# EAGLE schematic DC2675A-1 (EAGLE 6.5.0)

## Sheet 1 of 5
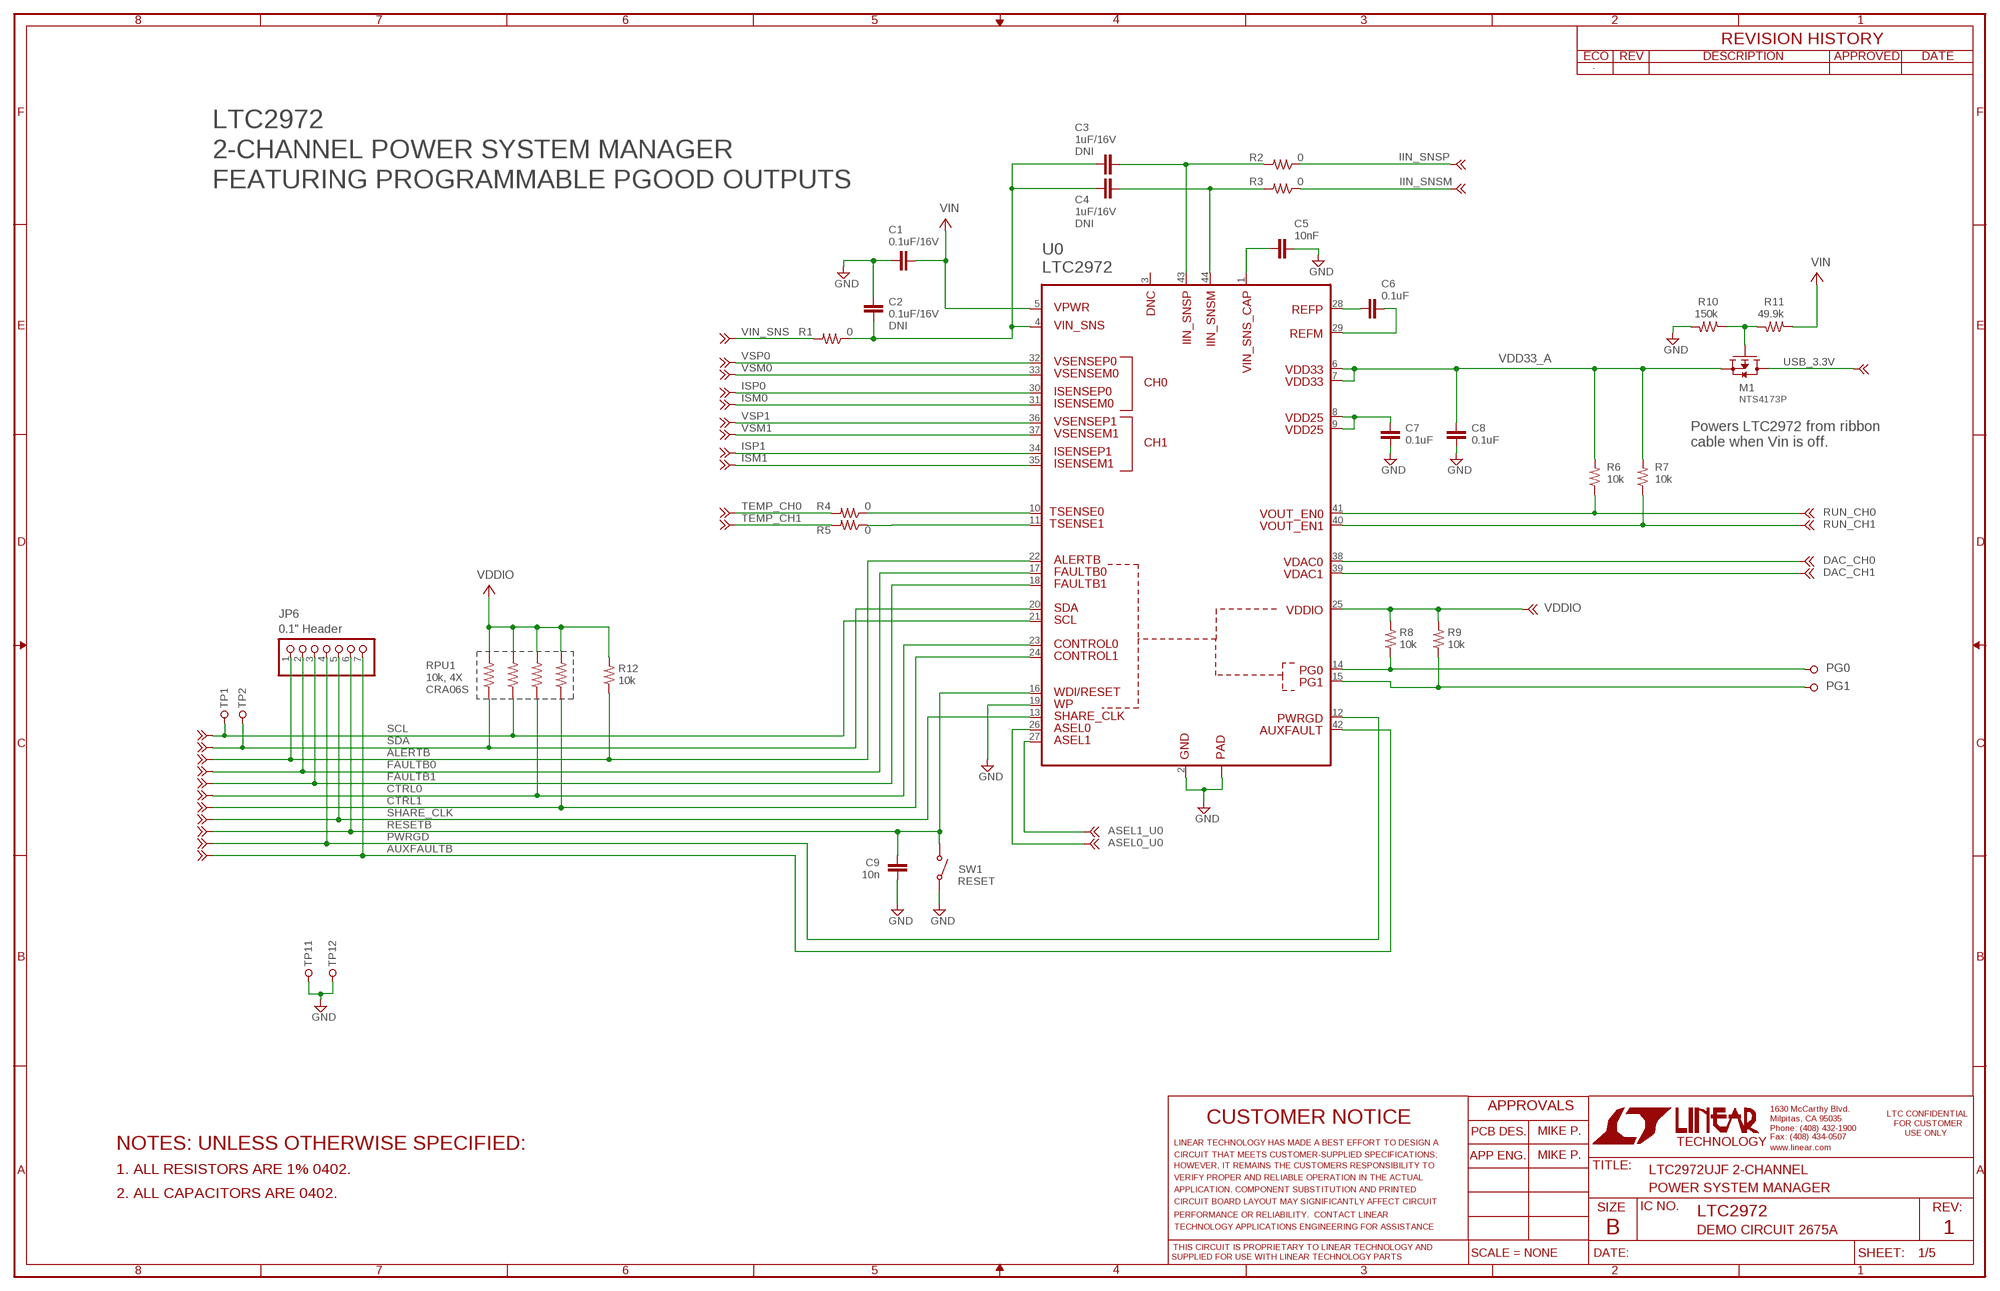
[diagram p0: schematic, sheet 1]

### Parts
C1  0.1uF/16V  CC0402  [C0402_BOX]
C2  0.1uF/16V  CC0402  [C0402_BOX]
C3  1uF/16V  CC0402  [C0402_BOX]
C4  1uF/16V  CC0402  [C0402_BOX]
C5  10nF  CC0402  [C0402_BOX]
C6  0.1uF  CC0402  [C0402_BOX]
C7  0.1uF  CC0402  [C0402_BOX]
C8  0.1uF  CC0402  [C0402_BOX]
C9  10n  CC0402  [C0402_BOX]
JP6  PINHD-1X7  [1X07]
M1  NTS4173P  PCH_SOT323  [SOT323]
R1  0  RR0402_BOX  [R0402_BOX]
R2  0  RR0402_BOX  [R0402_BOX]
R3  0  RR0402_BOX  [R0402_BOX]
R4  0  RR0402_BOX  [R0402_BOX]
R5  0  RR0402_BOX  [R0402_BOX]
R6  10k  RR0402_BOX  [R0402_BOX]
R7  10k  RR0402_BOX  [R0402_BOX]
R8  10k  RR0402_BOX  [R0402_BOX]
R9  10k  RR0402_BOX  [R0402_BOX]
R10  150k  RR0402_BOX  [R0402_BOX]
R11  49.9k  RR0402_BOX  [R0402_BOX]
R12  10k  RR0402_BOX  [R0402_BOX]
RPU1  10k, 4X  R_ARRAY_4X_CRA06S  [R_VISHAY_CRA06S]
SW1  PTS635SL25SMTR LFS  SWITCH_PTS635  [SWITCH_PTS635]
TP1  TURRET_SMALL_2308  [TURRET_SMALL_2308]
TP2  TURRET_SMALL_2308  [TURRET_SMALL_2308]
TP3  TURRET_SMALL_2308  [TURRET_SMALL_2308]
TP4  TURRET_SMALL_2308  [TURRET_SMALL_2308]
TP11  TURRET_SMALL_2308  [TURRET_SMALL_2308]
TP12  TURRET_SMALL_2308  [TURRET_SMALL_2308]
U0  LTC2972  [QFN44-6X7]

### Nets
ALERTB: JP6.1 R12.1 U0.22(ALERTB) ; also sheet 2,4,5
ASEL0_U0: U0.26(ASEL0) ; also sheet 3
ASEL1_U0: U0.27(ASEL1) ; also sheet 3
AUXFAULTB: JP6.7 U0.42(AUX_FAULT) ; also sheet 2,5
CTRL0: RPU1.R3_1 U0.23(CTRL0) ; also sheet 3,5
CTRL1: RPU1.R4_1 U0.24(CTRL1) ; also sheet 3,4,5
DAC_CH0: U0.38(VDAC0) ; also sheet 5
DAC_CH1: U0.39(VDAC1) ; also sheet 5
FAULTB0: JP6.2 U0.17(FAULTB0) ; also sheet 2,4,5
FAULTB1: JP6.3 U0.18(FAULTB1) ; also sheet 2,4,5
GND: C1.2 C2.1 C5.1 C7.2 C8.2 C9.1 R10.2 SW1.SW2 TP11.TP1 TP12.TP1 U0.2(GND) U0.19(WP) U0.45(PAD) ; also sheet 2,3,4,5
IIN_SNSM: R3.1 ; also sheet 5
IIN_SNSP: R2.1 ; also sheet 5
ISM0: U0.31(ISENSEM0) ; also sheet 3
ISM1: U0.35(ISENSEM1) ; also sheet 3
ISP0: U0.30(ISENSEP0) ; also sheet 3
ISP1: U0.34(ISENSEP1) ; also sheet 3
N$1: R4.1 U0.10(TSENSE0)
N$2: R5.1 U0.11(TSENSE1)
N$14: C2.2 C3.1 C4.1 R1.1 U0.4(VIN_SNS)
N$15: C3.2 R2.2 U0.43(IIN_SNSP)
N$16: C4.2 R3.2 U0.44(IIN_SNSM)
N$20: C5.2 U0.1(VIN_SNS_CAP)
N$48: C6.1 U0.28(REFP)
N$49: C6.2 U0.29(REFM)
N$52: C7.1 U0.8(VDD25) U0.9(VDD25)
PFET_GATE: M1.1(G) R10.1 R11.2 ; also sheet 2
PG0: R8.1 TP3.TP1 U0.14(PG0) ; also sheet 4
PG1: R9.1 TP4.TP1 U0.15(PG1) ; also sheet 4
PWRGD: JP6.4 U0.12(PWRGD) ; also sheet 2
RESETB: C9.2 JP6.6 SW1.SW1 U0.16(WDI-RESET) ; also sheet 2,5
RUN_CH0: R6.1 U0.41(VOUT_EN0) ; also sheet 5
RUN_CH1: R7.1 U0.40(VOUT_EN1) ; also sheet 5
SCL: RPU1.R2_1 TP1.TP1 U0.21(SCL) ; also sheet 2,5
SDA: RPU1.R1_1 TP2.TP1 U0.20(SDA) ; also sheet 2,5
SHARE_CLK: JP6.5 U0.13(SHARE_CLK) ; also sheet 2,5
TEMP_CH0: R4.2 ; also sheet 5
TEMP_CH1: R5.2 ; also sheet 5
USB_3.3V: M1.3(D) ; also sheet 2,5
VDD33_A: C8.1 M1.2(S) R6.2 R7.2 U0.6(VDD33) U0.7(VDD33) ; also sheet 3,4
VDDIO: R8.2 R9.2 R12.2 RPU1.R1_2 RPU1.R2_2 RPU1.R3_2 RPU1.R4_2 U0.25(VDDIO) ; also sheet 2,3,5
VIN: C1.1 R11.1 U0.5(VPWR) ; also sheet 2,5
VIN_SNS: R1.2 ; also sheet 2,5
VSM0: U0.33(VSENSEM0) ; also sheet 3
VSM1: U0.37(VSENSEM1) ; also sheet 3
VSP0: U0.32(VSENSEP0) ; also sheet 3
VSP1: U0.36(VSENSEP1) ; also sheet 3
Unconnected: U0.3(DNC)

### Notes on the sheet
- LTC2972
- 2-CHANNEL POWER SYSTEM MANAGER | DNI
- FEATURING PROGRAMMABLE PGOOD OUTPUTS
- DNI
- DNI
- Powers LTC2972 from ribbon
  cable when Vin is off.
- 0.1" Header
- CRA06S
- RESET
- MIKE P.
- NOTES: UNLESS OTHERWISE SPECIFIED:
- MIKE P.
- 1. ALL RESISTORS ARE 1% 0402. | LTC2972UJF 2-CHANNEL
- POWER SYSTEM MANAGER
- 2. ALL CAPACITORS ARE 0402.
- LTC2972
- DEMO CIRCUIT 2675A | 1

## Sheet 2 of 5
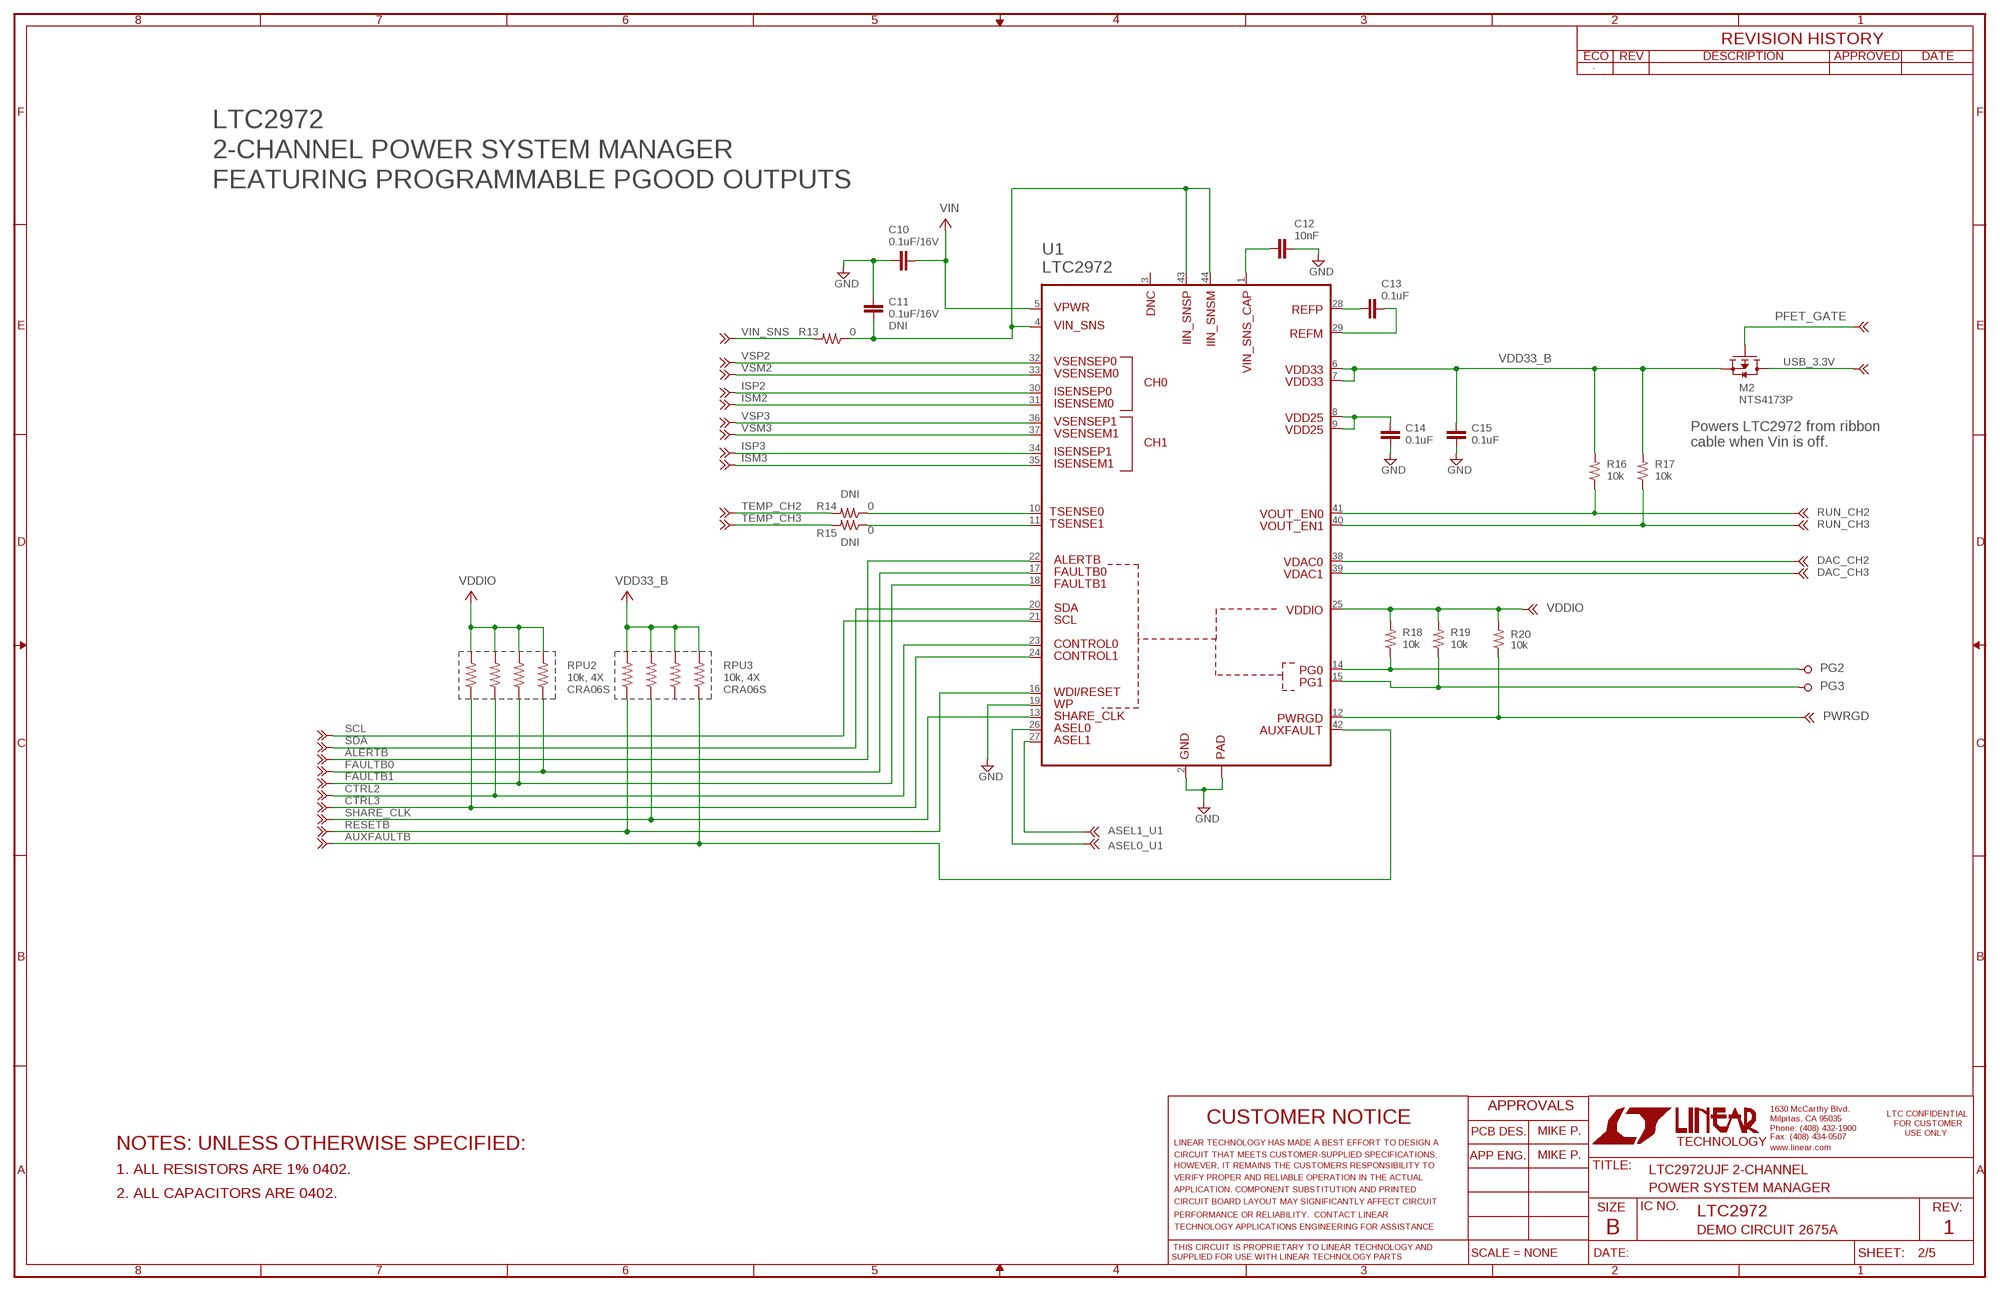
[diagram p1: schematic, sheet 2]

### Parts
C10  0.1uF/16V  CC0402  [C0402_BOX]
C11  0.1uF/16V  CC0402  [C0402_BOX]
C12  10nF  CC0402  [C0402_BOX]
C13  0.1uF  CC0402  [C0402_BOX]
C14  0.1uF  CC0402  [C0402_BOX]
C15  0.1uF  CC0402  [C0402_BOX]
M2  NTS4173P  PCH_SOT323  [SOT323]
R13  0  RR0402_BOX  [R0402_BOX]
R14  0  RR0402_BOX  [R0402_BOX]
R15  0  RR0402_BOX  [R0402_BOX]
R16  10k  RR0402_BOX  [R0402_BOX]
R17  10k  RR0402_BOX  [R0402_BOX]
R18  10k  RR0402_BOX  [R0402_BOX]
R19  10k  RR0402_BOX  [R0402_BOX]
R20  10k  RR0402_BOX  [R0402_BOX]
RPU2  10k, 4X  R_ARRAY_4X_CRA06S  [R_VISHAY_CRA06S]
RPU3  10k, 4X  R_ARRAY_4X_CRA06S  [R_VISHAY_CRA06S]
TP5  TURRET_SMALL_2308  [TURRET_SMALL_2308]
TP6  TURRET_SMALL_2308  [TURRET_SMALL_2308]
U1  LTC2972  [QFN44-6X7]

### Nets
ALERTB: U1.22(ALERTB) ; also sheet 1,4,5
ASEL0_U1: U1.26(ASEL0) ; also sheet 3
ASEL1_U1: U1.27(ASEL1) ; also sheet 3
AUXFAULTB: RPU3.R4_1 U1.42(AUX_FAULT) ; also sheet 1,5
CTRL2: RPU2.R2_1 U1.23(CTRL0) ; also sheet 3,4,5
CTRL3: RPU2.R1_1 U1.24(CTRL1) ; also sheet 3,4,5
DAC_CH2: U1.38(VDAC0) ; also sheet 5
DAC_CH3: U1.39(VDAC1) ; also sheet 5
FAULTB0: RPU2.R4_1 U1.17(FAULTB0) ; also sheet 1,4,5
FAULTB1: RPU2.R3_1 U1.18(FAULTB1) ; also sheet 1,4,5
GND: C10.2 C11.1 C12.1 C14.2 C15.2 U1.2(GND) U1.19(WP) U1.45(PAD) ; also sheet 1,3,4,5
ISM2: U1.31(ISENSEM0) ; also sheet 3
ISM3: U1.35(ISENSEM1) ; also sheet 3
ISP2: U1.30(ISENSEP0) ; also sheet 3
ISP3: U1.34(ISENSEP1) ; also sheet 3
N$4: R14.1 U1.10(TSENSE0)
N$5: R15.1 U1.11(TSENSE1)
N$17: C11.2 R13.1 U1.4(VIN_SNS) U1.43(IIN_SNSP) U1.44(IIN_SNSM)
N$24: C13.1 U1.28(REFP)
N$25: C13.2 U1.29(REFM)
N$26: C14.1 U1.8(VDD25) U1.9(VDD25)
N$27: C12.2 U1.1(VIN_SNS_CAP)
PFET_GATE: M2.1(G) ; also sheet 1
PG2: R18.1 TP5.TP1 U1.14(PG0) ; also sheet 4
PG3: R19.1 TP6.TP1 U1.15(PG1) ; also sheet 4
PWRGD: R20.1 U1.12(PWRGD) ; also sheet 1
RESETB: RPU3.R1_1 U1.16(WDI-RESET) ; also sheet 1,5
RUN_CH2: R16.1 U1.41(VOUT_EN0) ; also sheet 5
RUN_CH3: R17.1 U1.40(VOUT_EN1) ; also sheet 5
SCL: U1.21(SCL) ; also sheet 1,5
SDA: U1.20(SDA) ; also sheet 1,5
SHARE_CLK: RPU3.R2_1 U1.13(SHARE_CLK) ; also sheet 1,5
TEMP_CH2: R14.2 ; also sheet 5
TEMP_CH3: R15.2 ; also sheet 5
USB_3.3V: M2.3(D) ; also sheet 1,5
VDD33_B: C15.1 M2.2(S) R16.2 R17.2 RPU3.R1_2 RPU3.R2_2 RPU3.R3_2 RPU3.R4_2 U1.6(VDD33) U1.7(VDD33) ; also sheet 3,4,5
VDDIO: R18.2 R19.2 R20.2 RPU2.R1_2 RPU2.R2_2 RPU2.R3_2 RPU2.R4_2 U1.25(VDDIO) ; also sheet 1,3,5
VIN: C10.1 U1.5(VPWR) ; also sheet 1,5
VIN_SNS: R13.2 ; also sheet 1,5
VSM2: U1.33(VSENSEM0) ; also sheet 3
VSM3: U1.37(VSENSEM1) ; also sheet 3
VSP2: U1.32(VSENSEP0) ; also sheet 3
VSP3: U1.36(VSENSEP1) ; also sheet 3
Unconnected: RPU3.R3_1 U1.3(DNC)

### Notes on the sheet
- LTC2972
- 2-CHANNEL POWER SYSTEM MANAGER
- FEATURING PROGRAMMABLE PGOOD OUTPUTS
- DNI
- Powers LTC2972 from ribbon
  cable when Vin is off.
- DNI
- DNI
- CRA06S | CRA06S
- MIKE P.
- NOTES: UNLESS OTHERWISE SPECIFIED:
- MIKE P.
- 1. ALL RESISTORS ARE 1% 0402. | LTC2972UJF 2-CHANNEL
- POWER SYSTEM MANAGER
- 2. ALL CAPACITORS ARE 0402.
- LTC2972
- DEMO CIRCUIT 2675A | 1

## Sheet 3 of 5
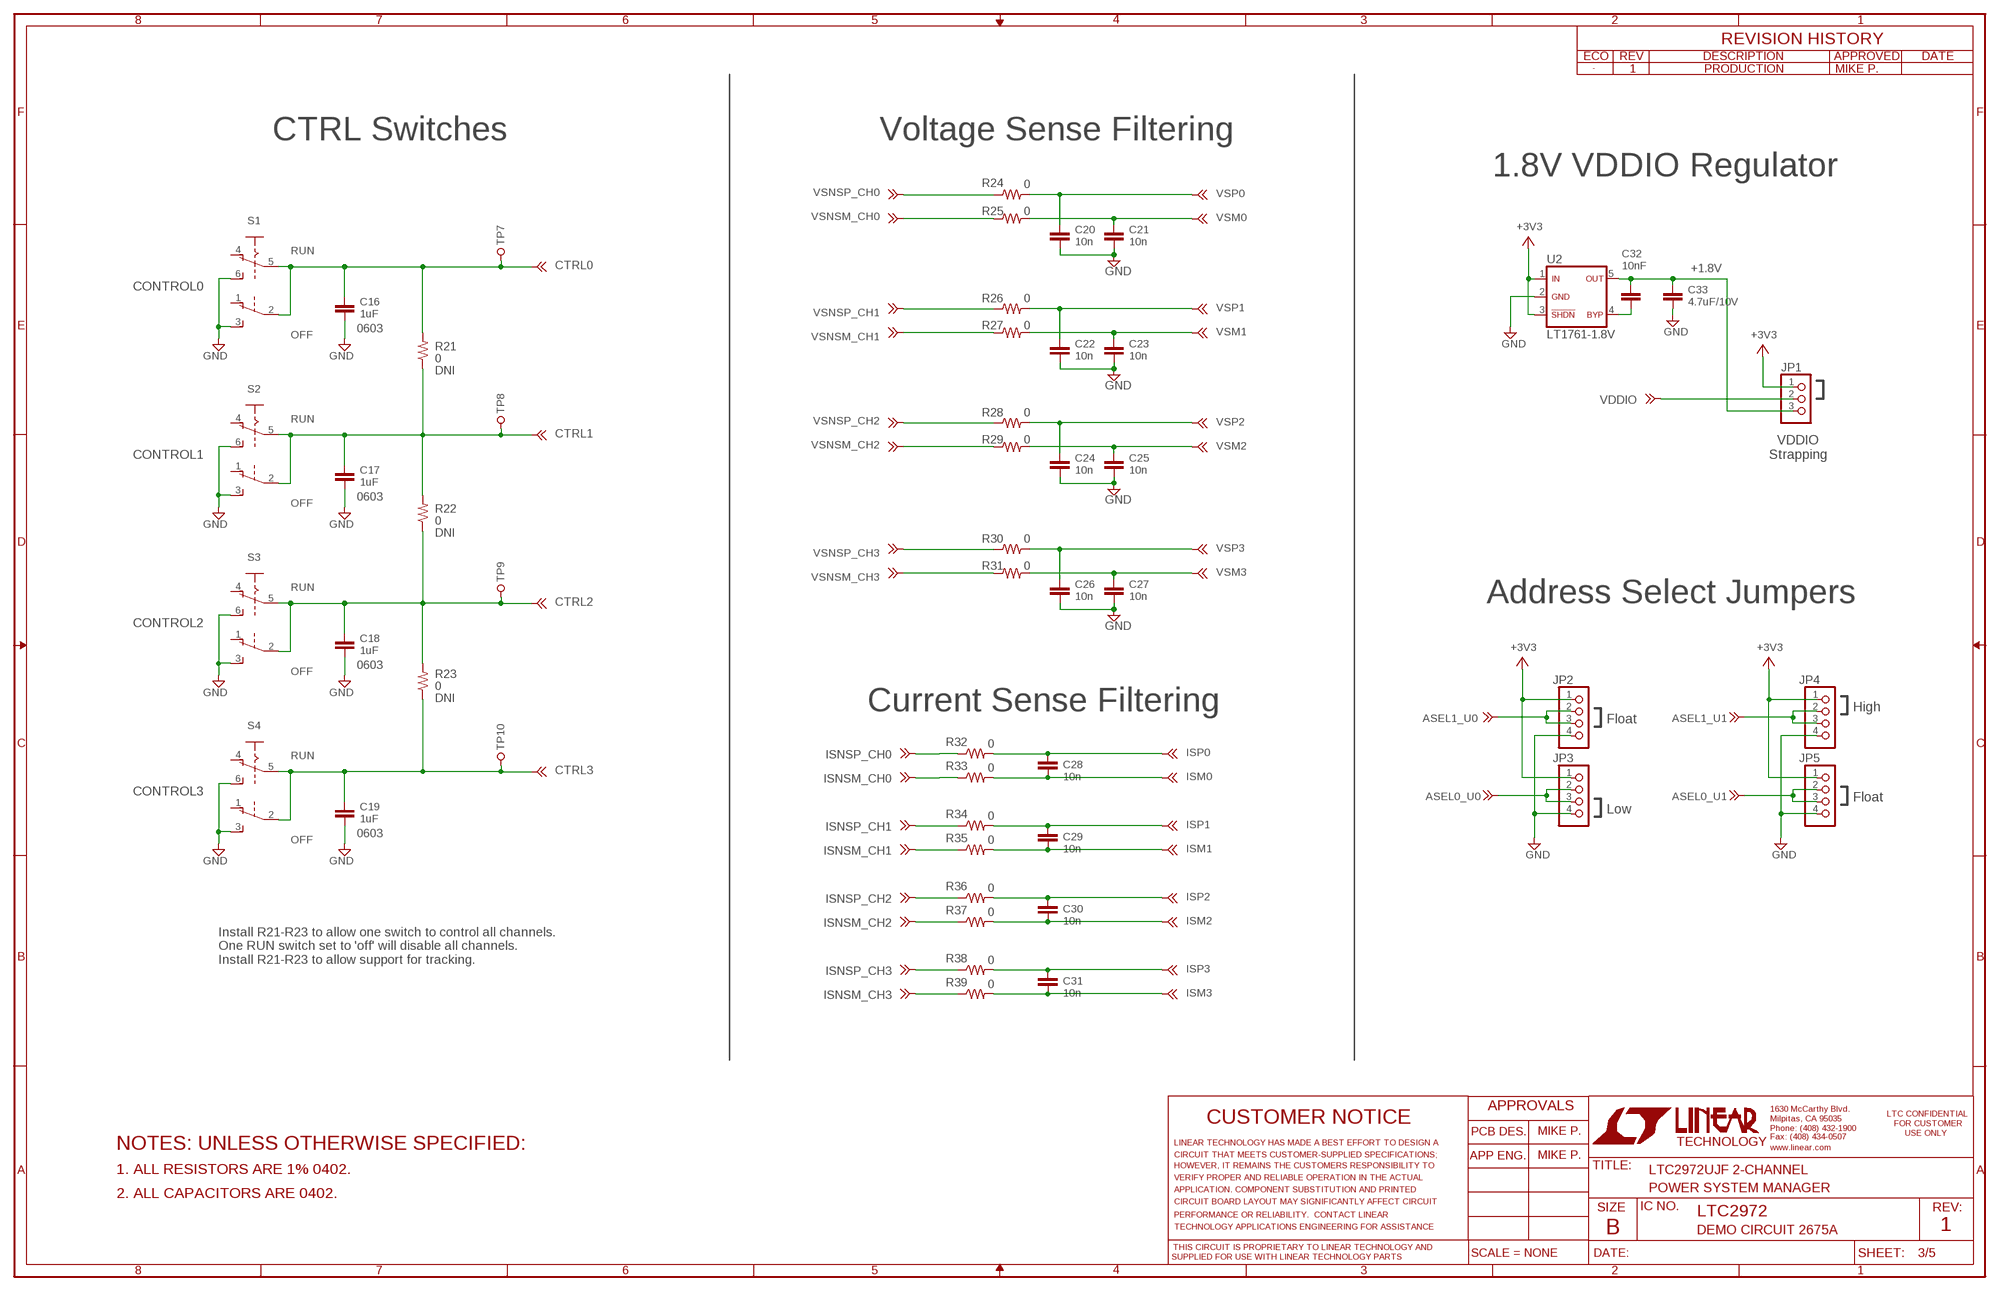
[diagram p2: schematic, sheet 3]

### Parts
C16  1uF  CC0603_BOX  [C0603_BOX]
C17  1uF  CC0603_BOX  [C0603_BOX]
C18  1uF  CC0603_BOX  [C0603_BOX]
C19  1uF  CC0603_BOX  [C0603_BOX]
C20  10n  CC0402  [C0402_BOX]
C21  10n  CC0402  [C0402_BOX]
C22  10n  CC0402  [C0402_BOX]
C23  10n  CC0402  [C0402_BOX]
C24  10n  CC0402  [C0402_BOX]
C25  10n  CC0402  [C0402_BOX]
C26  10n  CC0402  [C0402_BOX]
C27  10n  CC0402  [C0402_BOX]
C28  10n  CC0402  [C0402_BOX]
C29  10n  CC0402  [C0402_BOX]
C30  10n  CC0402  [C0402_BOX]
C31  10n  CC0402  [C0402_BOX]
C32  10nF  CC0402  [C0402_BOX]
C33  4.7uF/10V  CC0402  [C0402_BOX]
JP1  PINHD-1X3-2MM  [1X03-2MM]
JP2  PINHD-1X4-2MM  [1X04-2MM]
JP3  PINHD-1X4-2MM  [1X04-2MM]
JP4  PINHD-1X4-2MM  [1X04-2MM]
JP5  PINHD-1X4-2MM  [1X04-2MM]
R21  0  RR0402_BOX  [R0402_BOX]
R22  0  RR0402_BOX  [R0402_BOX]
R23  0  RR0402_BOX  [R0402_BOX]
R24  0  RR0402_BOX  [R0402_BOX]
R25  0  RR0402_BOX  [R0402_BOX]
R26  0  RR0402_BOX  [R0402_BOX]
R27  0  RR0402_BOX  [R0402_BOX]
R28  0  RR0402_BOX  [R0402_BOX]
R29  0  RR0402_BOX  [R0402_BOX]
R30  0  RR0402_BOX  [R0402_BOX]
R31  0  RR0402_BOX  [R0402_BOX]
R32  0  RR0402_BOX  [R0402_BOX]
R33  0  RR0402_BOX  [R0402_BOX]
R34  0  RR0402_BOX  [R0402_BOX]
R35  0  RR0402_BOX  [R0402_BOX]
R36  0  RR0402_BOX  [R0402_BOX]
R37  0  RR0402_BOX  [R0402_BOX]
R38  0  RR0402_BOX  [R0402_BOX]
R39  0  RR0402_BOX  [R0402_BOX]
S1  CONTROL0  JS202011CQN  [JS202011CQN]
S2  CONTROL1  JS202011CQN  [JS202011CQN]
S3  CONTROL2  JS202011CQN  [JS202011CQN]
S4  CONTROL3  JS202011CQN  [JS202011CQN]
TP7  TURRET_SMALL_2308  [TURRET_SMALL_2308]
TP8  TURRET_SMALL_2308  [TURRET_SMALL_2308]
TP9  TURRET_SMALL_2308  [TURRET_SMALL_2308]
TP10  TURRET_SMALL_2308  [TURRET_SMALL_2308]
U2  LT1761-1.8V  LT1761-X  [SOT-23-5]

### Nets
1V8: C32.1 C33.1 JP1.3 U2.5(OUT)
ASEL0_U0: JP3.2 JP3.3 ; also sheet 1
ASEL0_U1: JP5.2 JP5.3 ; also sheet 2
ASEL1_U0: JP2.2 JP2.3 ; also sheet 1
ASEL1_U1: JP4.2 JP4.3 ; also sheet 2
CTRL0: C16.1 R21.2 S1.2(B:P) S1.5(A:P) TP7.TP1 ; also sheet 1,5
CTRL1: C17.1 R21.1 R22.2 S2.2(B:P) S2.5(A:P) TP8.TP1 ; also sheet 1,4,5
CTRL2: C18.1 R22.1 R23.2 S3.2(B:P) S3.5(A:P) TP9.TP1 ; also sheet 2,4,5
CTRL3: C19.1 R23.1 S4.2(B:P) S4.5(A:P) TP10.TP1 ; also sheet 2,4,5
GND: C16.2 C17.2 C18.2 C19.2 C20.2 C21.2 C22.2 C23.2 C24.2 C25.2 C26.2 C27.2 C33.2 JP2.4 JP3.4 JP4.4 JP5.4 S1.3(B:S) S1.6(A:S) S2.3(B:S) S2.6(A:S) S3.3(B:S) S3.6(A:S) S4.3(B:S) S4.6(A:S) U2.2(GND) ; also sheet 1,2,4,5
ISM0: C28.2 R33.2 ; also sheet 1
ISM1: C29.2 R35.2 ; also sheet 1
ISM2: C30.2 R37.2 ; also sheet 2
ISM3: C31.2 R39.2 ; also sheet 2
ISNSM_CH0: R33.1 ; also sheet 5
ISNSM_CH1: R35.1 ; also sheet 5
ISNSM_CH2: R37.1 ; also sheet 5
ISNSM_CH3: R39.1 ; also sheet 5
ISNSP_CH0: R32.1 ; also sheet 5
ISNSP_CH1: R34.1 ; also sheet 5
ISNSP_CH2: R36.1 ; also sheet 5
ISNSP_CH3: R38.1 ; also sheet 5
ISP0: C28.1 R32.2 ; also sheet 1
ISP1: C29.1 R34.2 ; also sheet 1
ISP2: C30.1 R36.2 ; also sheet 2
ISP3: C31.1 R38.2 ; also sheet 2
N$34: C32.2 U2.4(BYP)
VDD33_A: JP1.1 JP2.1 JP3.1 U2.1(IN) U2.3(SHDN) ; supply symbol labelled +3V3 ; also sheet 1,4
VDD33_B: JP4.1 JP5.1 ; supply symbol labelled +3V3 ; also sheet 2,4,5
VDDIO: JP1.2 ; also sheet 1,2,5
VSM0: C21.1 R25.2 ; also sheet 1
VSM1: C23.1 R27.2 ; also sheet 1
VSM2: C25.1 R29.2 ; also sheet 2
VSM3: C27.1 R31.2 ; also sheet 2
VSNSM_CH0: R25.1 ; also sheet 5
VSNSM_CH1: R27.1 ; also sheet 5
VSNSM_CH2: R29.1 ; also sheet 5
VSNSM_CH3: R31.1 ; also sheet 5
VSNSP_CH0: R24.1 ; also sheet 5
VSNSP_CH1: R26.1 ; also sheet 5
VSNSP_CH2: R28.1 ; also sheet 5
VSNSP_CH3: R30.1 ; also sheet 5
VSP0: C20.1 R24.2 ; also sheet 1
VSP1: C22.1 R26.2 ; also sheet 1
VSP2: C24.1 R28.2 ; also sheet 2
VSP3: C26.1 R30.2 ; also sheet 2
Unconnected: S1.1(B:O) S1.4(A:O) S2.1(B:O) S2.4(A:O) S3.1(B:O) S3.4(A:O) S4.1(B:O) S4.4(A:O)

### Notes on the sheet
- 1 | PRODUCTION | MIKE P.
- CTRL Switches | Voltage Sense Filtering
- 1.8V VDDIO Regulator
- RUN
- +1.8V
- 0603
- OFF
- DNI
- RUN
- VDDIO
  Strapping
- 0603
- OFF
- DNI
- RUN
- Address Select Jumpers
- 0603
- OFF
- DNI
- Current Sense Filtering | High
- Float
- RUN
- Float
- Low
- 0603
- OFF
- Install R21-R23 to allow one switch to control all channels.
  One RUN switch set to 'off' will disable all channels.
  Install R21-R23 to allow support for tracking.
- MIKE P.
- NOTES: UNLESS OTHERWISE SPECIFIED:
- MIKE P.
- 1. ALL RESISTORS ARE 1% 0402. | LTC2972UJF 2-CHANNEL
- POWER SYSTEM MANAGER
- 2. ALL CAPACITORS ARE 0402.
- LTC2972
- DEMO CIRCUIT 2675A | 1

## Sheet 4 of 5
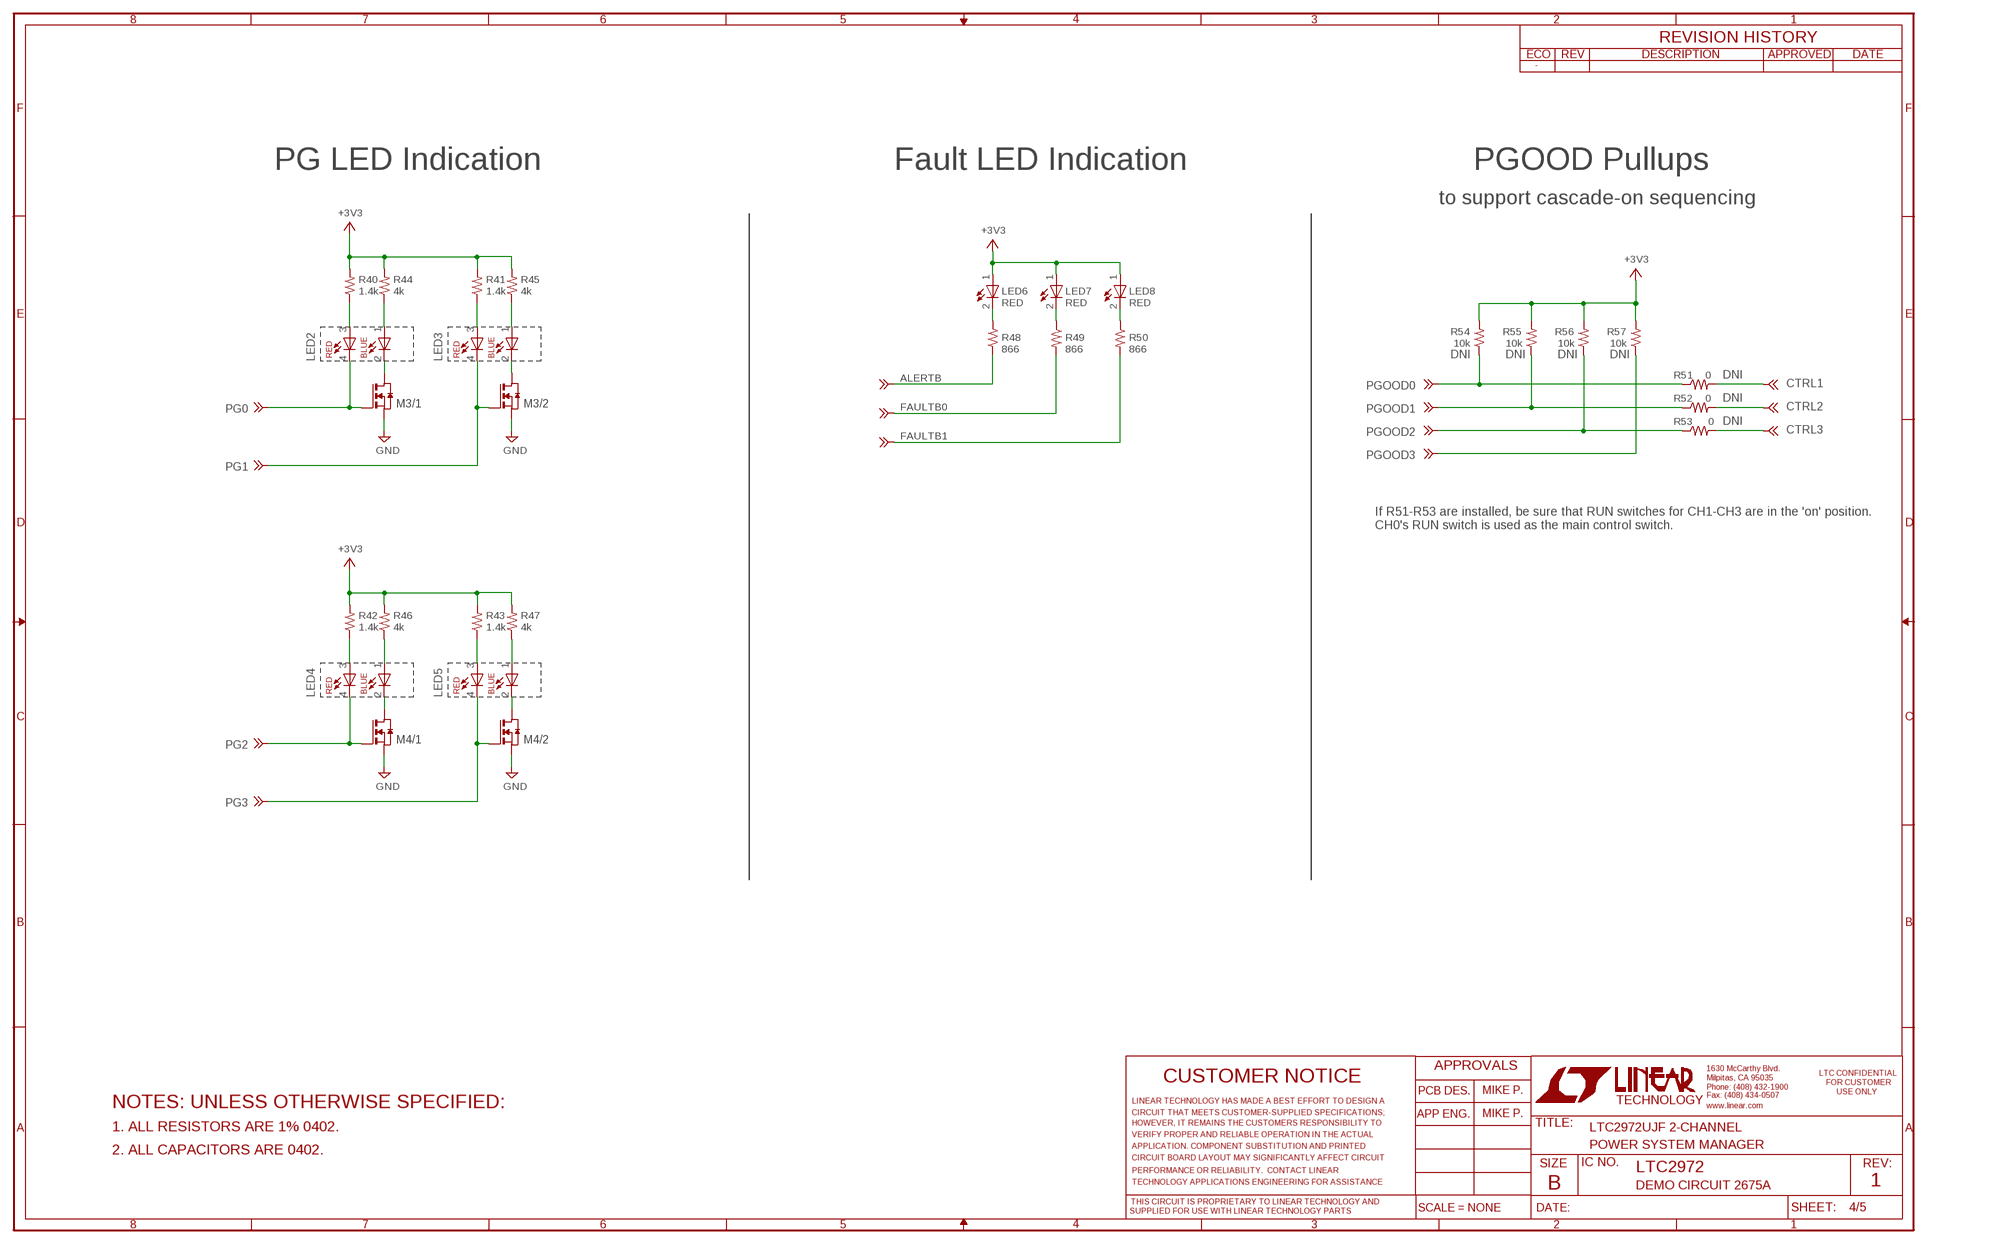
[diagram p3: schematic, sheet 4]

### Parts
LED2  Kingbright  LED-DUAL-COLOR_1.6X0.8MM  [LED-DUAL_1.6X0.8MM]
LED3  Kingbright  LED-DUAL-COLOR_1.6X0.8MM  [LED-DUAL_1.6X0.8MM]
LED4  Kingbright  LED-DUAL-COLOR_1.6X0.8MM  [LED-DUAL_1.6X0.8MM]
LED5  Kingbright  LED-DUAL-COLOR_1.6X0.8MM  [LED-DUAL_1.6X0.8MM]
LED6  RED  LED-0603  [CHIPLED_0603]
LED7  RED  LED-0603  [CHIPLED_0603]
LED8  RED  LED-0603  [CHIPLED_0603]
M3  NCH_DUAL_REVERSE  [SOT-363]
M4  NCH_DUAL_REVERSE  [SOT-363]
R40  1.4k  RR0402_BOX  [R0402_BOX]
R41  1.4k  RR0402_BOX  [R0402_BOX]
R42  1.4k  RR0402_BOX  [R0402_BOX]
R43  1.4k  RR0402_BOX  [R0402_BOX]
R44  4k  RR0402_BOX  [R0402_BOX]
R45  4k  RR0402_BOX  [R0402_BOX]
R46  4k  RR0402_BOX  [R0402_BOX]
R47  4k  RR0402_BOX  [R0402_BOX]
R48  866  RR0402_BOX  [R0402_BOX]
R49  866  RR0402_BOX  [R0402_BOX]
R50  866  RR0402_BOX  [R0402_BOX]
R51  0  RR0402_BOX  [R0402_BOX]
R52  0  RR0402_BOX  [R0402_BOX]
R53  0  RR0402_BOX  [R0402_BOX]
R54  10k  RR0402_BOX  [R0402_BOX]
R55  10k  RR0402_BOX  [R0402_BOX]
R56  10k  RR0402_BOX  [R0402_BOX]
R57  10k  RR0402_BOX  [R0402_BOX]

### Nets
ALERTB: R48.1 ; also sheet 1,2,5
CTRL1: R51.2 ; also sheet 1,3,5
CTRL2: R52.2 ; also sheet 2,3,5
CTRL3: R53.2 ; also sheet 2,3,5
FAULTB0: R49.2 ; also sheet 1,2,5
FAULTB1: R50.2 ; also sheet 1,2,5
GND: M3.1(/1:S) M3.4(/2:S) M4.1(/1:S) M4.4(/2:S) ; also sheet 1,2,3,5
N$8: LED5.2(C2) M4.3(/2:D)
N$9: LED4.2(C2) M4.6(/1:D)
N$10: LED2.2(C2) M3.6(/1:D)
N$11: LED3.2(C2) M3.3(/2:D)
N$12: LED2.1(A1) R44.1
N$13: LED3.1(A1) R45.1
N$18: LED4.1(A1) R46.1
N$19: LED5.1(A1) R47.1
N$28: LED8.N(C) R50.1
N$29: LED7.N(C) R49.1
N$30: LED6.N(C) R48.2
N$36: LED2.3(A3) R40.1
N$42: LED3.3(A3) R41.1
N$56: LED4.3(A3) R42.1
N$83: LED5.3(A3) R43.1
PG0: LED2.4(C4) M3.2(/1:G) ; also sheet 1
PG1: LED3.4(C4) M3.5(/2:G) ; also sheet 1
PG2: LED4.4(C4) M4.2(/1:G) ; also sheet 2
PG3: LED5.4(C4) M4.5(/2:G) ; also sheet 2
PGOOD0: R51.1 R54.1 ; also sheet 5
PGOOD1: R52.1 R55.1 ; also sheet 5
PGOOD2: R53.1 R56.1 ; also sheet 5
PGOOD3: R57.1 ; also sheet 5
VDD33_A: R40.2 R41.2 R44.2 R45.2 ; supply symbol labelled +3V3 ; also sheet 1,3
VDD33_B: LED6.P(A) LED7.P(A) LED8.P(A) R42.2 R43.2 R46.2 R47.2 R54.2 R55.2 R56.2 R57.2 ; supply symbol labelled +3V3 ; also sheet 2,3,5

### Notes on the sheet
- PG LED Indication | Fault LED Indication | PGOOD Pullups
- to support cascade-on sequencing
- DNI | DNI | DNI | DNI
- DNI
- DNI
- DNI
- If R51-R53 are installed, be sure that RUN switches for CH1-CH3 are in the 'on' position.
  CH0's RUN switch is used as the main control switch.
- MIKE P.
- NOTES: UNLESS OTHERWISE SPECIFIED:
- MIKE P.
- 1. ALL RESISTORS ARE 1% 0402. | LTC2972UJF 2-CHANNEL
- POWER SYSTEM MANAGER
- 2. ALL CAPACITORS ARE 0402.
- LTC2972
- DEMO CIRCUIT 2675A | 1

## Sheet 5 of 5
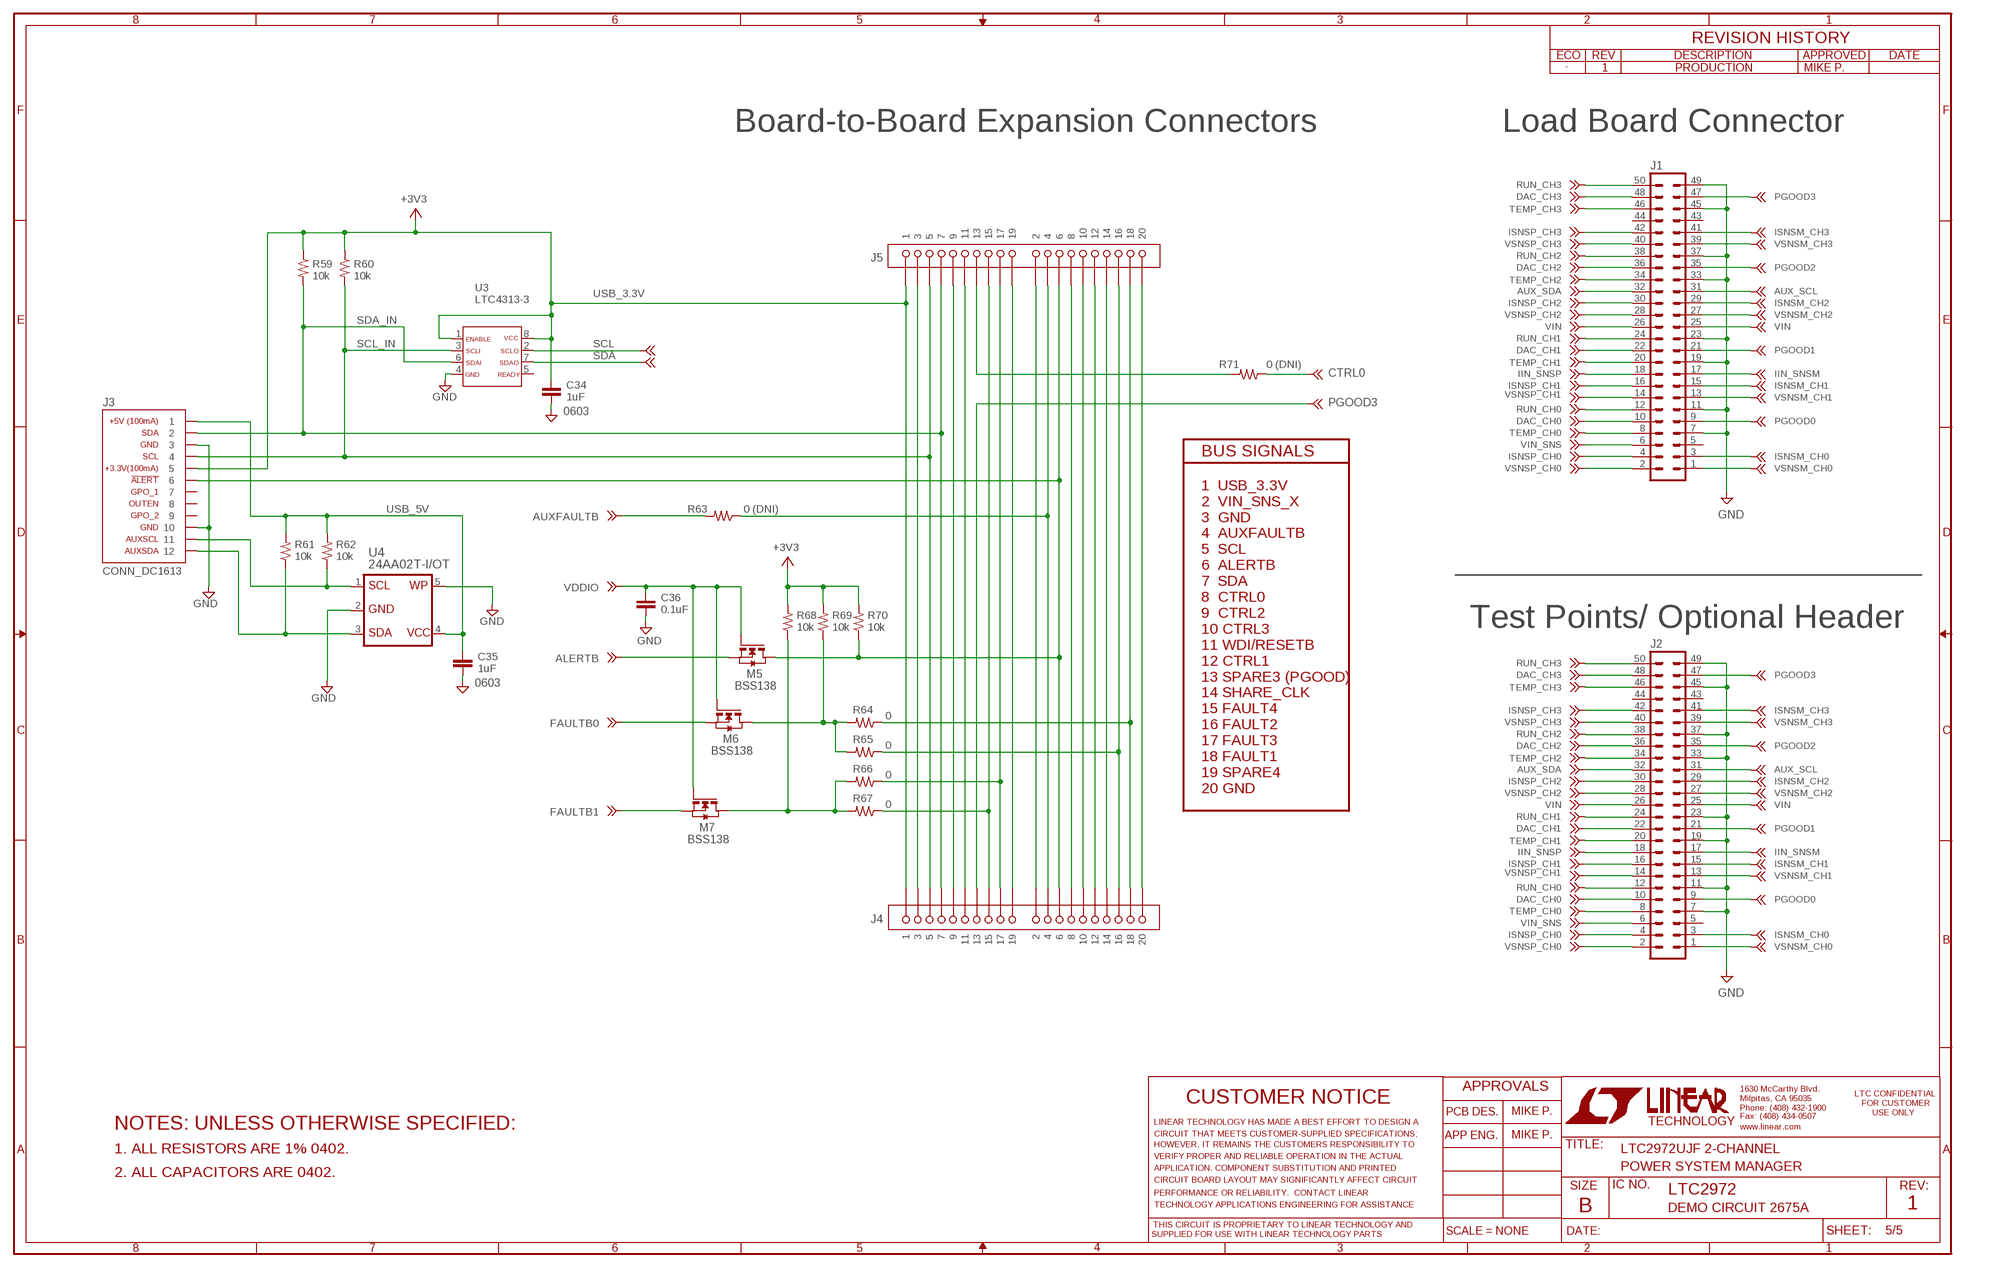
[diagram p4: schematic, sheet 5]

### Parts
C34  1uF  CC0603_BOX  [C0603_BOX]
C35  1uF  CC0603_BOX  [C0603_BOX]
C36  0.1uF  CC0402  [C0402_BOX]
J1  CONN_2X25_RECEPT  [PINHEAD_2X25_RECEPT]
J2  CONN_2X25_RECEPT_NO_SILK  [PINHEAD_2X25_RECEPT_NO_SILK]
J3  CONN_DC1613  [CONN_DC1613]
J4  HEADER_CONN_2X10_0.1INCH  [HEADER_2X10_0.1INCH]
J5  RECEPT_CONN_2X10_0.1INCH  [RECEPT_2X10_0.1INCH]
M5  BSS138  NCH_SOT23  [SOT23]
M6  BSS138  NCH_SOT23  [SOT23]
M7  BSS138  NCH_SOT23  [SOT23]
R59  10k  RR0402_BOX  [R0402_BOX]
R60  10k  RR0402_BOX  [R0402_BOX]
R61  10k  RR0402_BOX  [R0402_BOX]
R62  10k  RR0402_BOX  [R0402_BOX]
R63  0 (DNI)  RR0402_BOX  [R0402_BOX]
R64  0  RR0402_BOX  [R0402_BOX]
R65  0  RR0402_BOX  [R0402_BOX]
R66  0  RR0402_BOX  [R0402_BOX]
R67  0  RR0402_BOX  [R0402_BOX]
R68  10k  RR0402_BOX  [R0402_BOX]
R69  10k  RR0402_BOX  [R0402_BOX]
R70  10k  RR0402_BOX  [R0402_BOX]
R71  0 (DNI)  RR0402_BOX  [R0402_BOX]
U3  LTC4313-3  LTC4313_MS8  [MSOP-8]
U4  24AA02T-I/OT  24AA64  [SOT-23-5]

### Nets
ALERTB: M5.2(S) ; also sheet 1,2,4
ALERTB_3V3: J3.6 J4.P$6 J5.P$6 M5.3(D) R70.1
AUX_SCL: J1.31 J2.31 J3.11 R62.1 U4.1
AUX_SDA: J1.32 J2.32 J3.12 R61.1 U4.3
AUXFAULTB: R63.2 ; also sheet 1,2
AUXFAULTB_3V3: J4.P$4 J5.P$4 R63.1
CTRL0: J4.P$8 J5.P$8 R71.1 ; also sheet 1,3
CTRL1: J4.P$12 J5.P$12 ; also sheet 1,3,4
CTRL2: J4.P$9 J5.P$9 ; also sheet 2,3,4
CTRL3: J4.P$10 J5.P$10 ; also sheet 2,3,4
DAC_CH0: J1.10 J2.10 ; also sheet 1
DAC_CH1: J1.22 J2.22 ; also sheet 1
DAC_CH2: J1.36 J2.36 ; also sheet 2
DAC_CH3: J1.48 J2.48 ; also sheet 2
FAULT1: J4.P$18 J5.P$18 R64.1
FAULT2: J4.P$16 J5.P$16 R65.1
FAULT3: J4.P$17 J5.P$17 R66.1
FAULT4: J4.P$15 J5.P$15 R67.1
FAULTB0: M6.2(S) ; also sheet 1,2,4
FAULTB1: M7.2(S) ; also sheet 1,2,4
GND: C34.2 C35.2 C36.2 J1.7 J1.11 J1.19 J1.23 J1.33 J1.37 J1.45 J1.49 J2.7 J2.11 J2.19 J2.23 J2.33 J2.37 J2.45 J2.49 J3.3 J3.10 J4.P$3 J4.P$20 J5.P$3 J5.P$20 U3.4(GND) U4.2 U4.5 ; also sheet 1,2,3,4
IIN_SNSM: J1.17 J2.17 ; also sheet 1
IIN_SNSP: J1.18 J2.18 ; also sheet 1
ISNSM_CH0: J1.3 J2.3 ; also sheet 3
ISNSM_CH1: J1.15 J2.15 ; also sheet 3
ISNSM_CH2: J1.29 J2.29 ; also sheet 3
ISNSM_CH3: J1.41 J2.41 ; also sheet 3
ISNSP_CH0: J1.4 J2.4 ; also sheet 3
ISNSP_CH1: J1.16 J2.16 ; also sheet 3
ISNSP_CH2: J1.30 J2.30 ; also sheet 3
ISNSP_CH3: J1.42 J2.42 ; also sheet 3
N$6: J5.P$13 R71.2
N$21: M7.3(D) R66.2 R67.2 R68.1
N$23: M6.3(D) R64.2 R65.2 R69.1
PGOOD0: J1.9 J2.9 ; also sheet 4
PGOOD1: J1.21 J2.21 ; also sheet 4
PGOOD2: J1.35 J2.35 ; also sheet 4
PGOOD3: J1.47 J2.47 J4.P$13 ; also sheet 4
RESETB: J4.P$11 J5.P$11 ; also sheet 1,2
RUN_CH0: J1.12 J2.12 ; also sheet 1
RUN_CH1: J1.24 J2.24 ; also sheet 1
RUN_CH2: J1.38 J2.38 ; also sheet 2
RUN_CH3: J1.50 J2.50 ; also sheet 2
SCL: U3.2(SCLO) ; also sheet 1,2
SCL_IN: J3.4 J4.P$5 J5.P$5 R60.2 U3.3(SCLI)
SDA: U3.7(SDAO) ; also sheet 1,2
SDA_IN: J3.2 J4.P$7 J5.P$7 R59.2 U3.6(SDAI)
SHARE_CLK: J4.P$14 J5.P$14 ; also sheet 1,2
SPARE4: J4.P$19 J5.P$19
TEMP_CH0: J1.8 J2.8 ; also sheet 1
TEMP_CH1: J1.20 J2.20 ; also sheet 1
TEMP_CH2: J1.34 J2.34 ; also sheet 2
TEMP_CH3: J1.46 J2.46 ; also sheet 2
USB_3.3V: C34.1 J3.5 J4.P$1 J5.P$1 R59.1 R60.1 U3.1(EN) U3.8(VCC) ; supply symbol labelled +3V3 ; also sheet 1,2
USB_5V: C35.1 J3.1 R61.2 R62.2 U4.4
VDD33_B: R68.2 R69.2 R70.2 ; supply symbol labelled +3V3 ; also sheet 2,3,4
VDDIO: C36.1 M5.1(G) M6.1(G) M7.1(G) ; also sheet 1,2,3
VIN: J1.25 J1.26 J2.25 J2.26 ; also sheet 1,2
VIN_SNS: J1.6 J2.6 ; also sheet 1,2
VIN_SNS_X: J4.P$2 J5.P$2
VSNSM_CH0: J1.1 J2.1 ; also sheet 3
VSNSM_CH1: J1.13 J2.13 ; also sheet 3
VSNSM_CH2: J1.27 J2.27 ; also sheet 3
VSNSM_CH3: J1.39 J2.39 ; also sheet 3
VSNSP_CH0: J1.2 J2.2 ; also sheet 3
VSNSP_CH1: J1.14 J2.14 ; also sheet 3
VSNSP_CH2: J1.28 J2.28 ; also sheet 3
VSNSP_CH3: J1.40 J2.40 ; also sheet 3
Unconnected: J1.5 J1.43 J1.44 J2.5 J2.43 J2.44 J3.7 J3.8 J3.9 U3.5(RDY)

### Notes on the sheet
- 1 | PRODUCTION | MIKE P.
- Board-to-Board Expansion Connectors | Load Board Connector
- 0603
- VIN_SNS
- BUS SIGNALS
- Test Points/ Optional Header
- 0603
- 1  USB_3.3V
  2  VIN_SNS_X
  3  GND
  4  AUXFAULTB
  5  SCL
  6  ALERTB
  7  SDA
  8  CTRL0
  9  CTRL2
  10 CTRL3
  11 WDI/RESETB
  12 CTRL1
  13 SPARE3 (PGOOD)
  14 SHARE_CLK
  15 FAULT4
  16 FAULT2
  17 FAULT3
  18 FAULT1
  19 SPARE4
  20 GND
- VIN_SNS
- MIKE P.
- NOTES: UNLESS OTHERWISE SPECIFIED:
- MIKE P.
- 1. ALL RESISTORS ARE 1% 0402. | LTC2972UJF 2-CHANNEL
- POWER SYSTEM MANAGER
- 2. ALL CAPACITORS ARE 0402.
- LTC2972
- DEMO CIRCUIT 2675A | 1

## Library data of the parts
C1-C36 = rcl:C: CAPACITOR, European symbol
J1 = con-sullinselectronics:CONN_2X25_RECEPT
J2 = con-sullinselectronics:CONN_2X25_RECEPT_NO_SILK
J3 = con-fci:CONN_DC1613: Connector for LT DC1613 USB Dongle
J4 = con-millmax:HEADER_CONN_2X10_0.1INCH
J5 = con-millmax:RECEPT_CONN_2X10_0.1INCH
JP1 = pinhead:PINHD-1X3-2MM: PIN HEADER
JP2-JP5 = pinhead:PINHD-1X4-2MM: PIN HEADER
JP6 = pinhead:PINHD-1X7: PIN HEADER
LED2-LED5 = led:LED-DUAL-COLOR_1.6X0.8MM
LED6-LED8 = led:LED-0603: SMD LED in R0603
M1 M2 = transistor-fet:PCH_
M3 M4 = transistor-fet:NCH_DUAL_REVERSE
M5-M7 = transistor-fet:NCH_
R1-R57 R59-R71 = resistor:R: RESISTOR, American symbol
RPU1-RPU3 = kalin:R_ARRAY_4X_CRA06S: Thick Film Resistor Array
S1-S4 = kalin:JS202011CQN: SLIDING SWITCH Siemens, distributor Buerklin, 11G766
SW1 = kalin:SWITCH_PTS635: PTS635SL25 Surface Mount Tactile Switch
TP1-TP12 = testpad:TURRET_SMALL_2308: Small Test Turret Mill-Max 2308
U0 U1 = linear-technology:LTC2972
U2 = linear-technology:LT1761-X: 100mA, Low Noise, Fixed LDO Micropower Regulators w/ SHDN in TSOT-23
U3 = linear-technology:LTC4313: 2-Wire Bus Buffers with High Noise Margin
U4 = kalin:24AA64: 64Kbit I2C Serial EEPROM in SOT-23-5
